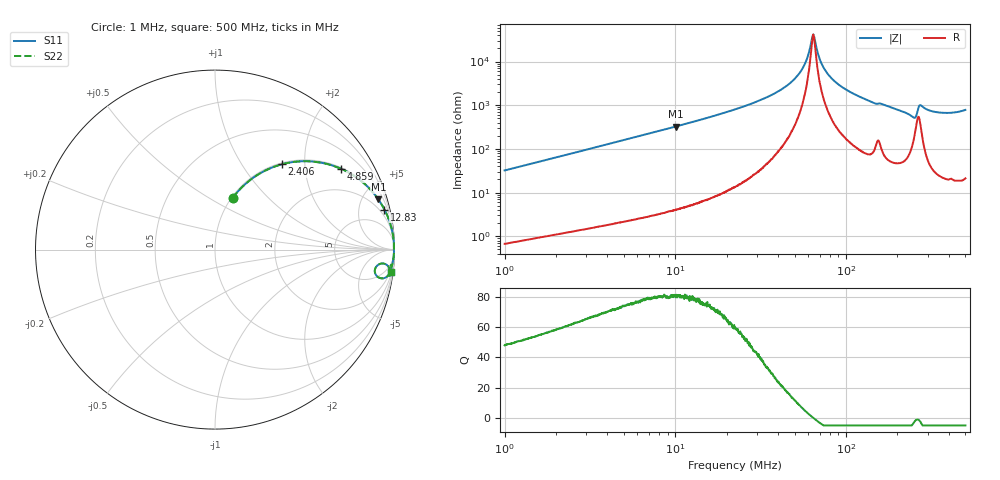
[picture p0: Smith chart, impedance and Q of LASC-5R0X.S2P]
!s-Parameter Generated by FASTRON Sdn. Bhd.
!FASTRON P/N : LASC-5R0X
!Keysight Technologies,E4991B,MY54100416,A.01.15
!Date: Thu Mar 12 10:17:13 2026
!Version  : Rev00 Thu Mar 12 10:17:13 2026
!Data & Calibration Information:
!PortZ  Port1:50+j0  Port2:50+j0
!When reading, reference impedance value at option line is always used.
!Remarks : This data is being provided solely for informational purposes.
!Freq	S11	S21	S12	S22
# Hz S dB R 50
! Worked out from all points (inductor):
!   1601 points, 1 MHz to 500 MHz, reference 50 ohm
!   read as one part in series: L = 5.1 uH near 1.032 MHz
!   highest Q = 80.9 at 10.05 MHz (marker M1), where L = 5.15 uH
!   self-resonance near 64.07 MHz
!   S11 on the Smith chart (normalised r, x): 1 MHz: 1.01, +0.64; 2.406 MHz: 1.03, +1.53; 4.859 MHz: 1.04, +3.10; 12.83 MHz: 1.11, +8.43; 500 MHz: 1, -16
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1000000  -10.33 71.1  -0.48 -17.7  -0.48 -17.7  -10.33 71.1
2405634  -4.38 51.9  -2.08 -37.1  -2.08 -37.1  -4.38 51.9
2820919  -3.57 47.6  -2.64 -41.5  -2.64 -41.5  -3.57 47.6
4859040  -1.57 32.6  -5.36 -56.6  -5.36 -56.6  -1.57 32.6
7957584  -0.66 21.3  -8.79 -68.0  -8.79 -68.0  -0.66 21.3
1.004599e7  -0.42 17.0  -10.66 -72.2  -10.66 -72.2  -0.42 17.0
1.283112e7  -0.26 13.3  -12.76 -76.0  -12.76 -76.0  -0.26 13.3
2.236068e7  -0.08 7.1  -18.17 -82.0  -18.17 -82.0  -0.08 7.1
3.563754e7  -0.03 3.5  -24.26 -84.7  -24.26 -84.7  -0.03 3.5
4.7875e7  -0.02 1.7  -30.68 -84.1  -30.68 -84.1  -0.02 1.7
5.657749e7  -0.02 0.7  -37.93 -78.9  -37.93 -78.9  -0.02 0.7
6.307767e7  -0.02 0.1  -50.42 -37.4  -50.42 -37.4  -0.02 0.1
6.532168e7  -0.02 -0.1  -50.70 31.9  -50.70 31.9  -0.02 -0.1
6.978047e7  -0.02 -0.5  -41.50 71.9  -41.50 71.9  -0.02 -0.5
7.425464e7  -0.02 -0.8  -36.92 78.4  -36.92 78.4  -0.02 -0.8
8.707324e7  -0.03 -1.7  -30.52 82.8  -30.52 82.8  -0.03 -1.7
1.197311e8  -0.05 -3.6  -24.00 82.9  -24.00 82.9  -0.05 -3.6
1.77937e8  -0.10 -6.1  -19.46 80.5  -19.46 80.5  -0.10 -6.1
2.475421e8  -0.57 -9.8  -15.04 64.2  -15.04 64.2  -0.57 -9.8
2.738466e8  -0.31 -5.3  -20.27 66.0  -20.27 66.0  -0.31 -5.3
3.538668e8  -0.14 -8.3  -16.77 79.7  -16.77 79.7  -0.14 -8.3
5e8  -0.10 -7.3  -17.97 81.2  -17.97 81.2  -0.10 -7.3
